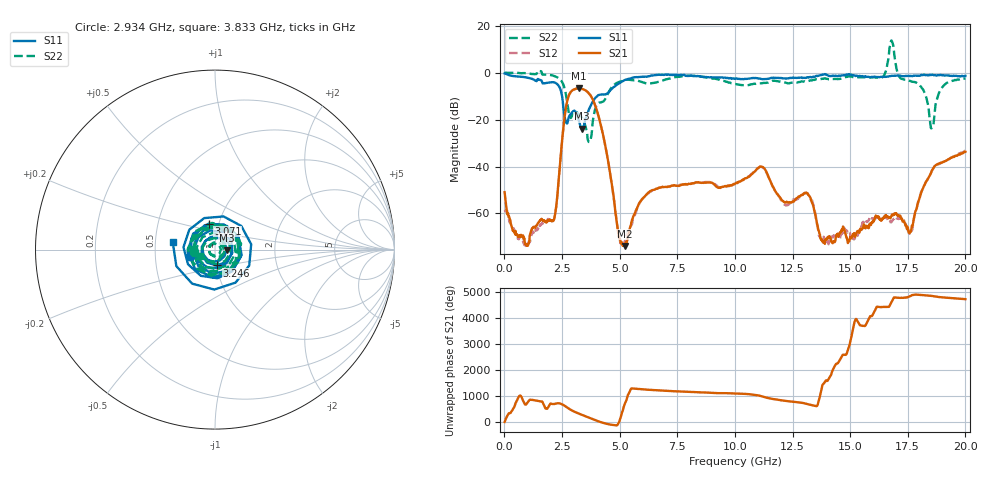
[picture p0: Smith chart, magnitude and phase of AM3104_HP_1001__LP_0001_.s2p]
!Created with skrf (http://scikit-rf.org).
# Hz S RI R 50.0
!freq ReS11 ImS11 ReS21 ImS21 ReS12 ImS12 ReS22 ImS22
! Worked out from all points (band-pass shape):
!   1601 points, 10 MHz to 20 GHz, reference 50 ohm
!   highest |S21| = -6.73 dB at 3.246 GHz (marker M1); lowest = -73.8 dB at 5.22 GHz (marker M2)
!   |S21| within 3 dB of the highest: 2.796 GHz to 3.741 GHz (944.9 MHz wide, 28.9 % of centre)
!   lowest |S11| = -23.8 dB at 3.346 GHz (marker M3), VSWR 1.14, Z = 56.9 - j0.37 ohm
!   |S11| at or under -10 dB: 2.502 GHz to 4.029 GHz (1.527 GHz wide, 46.8 % of centre)
!   |S22| runs from -29.6 to 13.7 dB; largest |S21 - S12| = 0.024
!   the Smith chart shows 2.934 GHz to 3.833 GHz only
!   S11 on the Smith chart (normalised r, x): 2.934 GHz: 0.76, -0.06; 3.071 GHz: 0.89, +0.26; 3.246 GHz: 1.00, -0.18; 3.833 GHz: 0.62, +0.05
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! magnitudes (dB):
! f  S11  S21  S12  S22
! 10 MHz  -0.3  -50.9  -58.4  0.0
! 972 MHz  -2.1  -73.2  -73.7  -0.2
! 2.109 GHz  -4.1  -63.2  -63.1  -1.2
! 2.646 GHz  -20.3  -16.5  -16.5  -8.1
! 2.934 GHz  -16.9  -7.7  -7.7  -18.4
! 3.071 GHz  -16.5  -7.0  -7.0  -16.5
! 3.246 GHz  -21.0  -6.7  -6.8  -18.1
! 3.346 GHz  -23.8  -6.9  -7.0  -18.9
! 3.833 GHz  -12.4  -11.4  -11.4  -20.9
! 5.22 GHz  -3.2  -73.8  -72.1  -3.2
! 6.682 GHz  -0.9  -49.2  -49.1  -3.9
! 10.01 GHz  -2.6  -47.4  -47.6  -4.9
! 11.17 GHz  -2.8  -40.1  -40.2  -4.5
! 12.15 GHz  -2.5  -55.2  -56.3  -4.2
! 13.34 GHz  -2.0  -55.1  -54.4  -3.3
! 13.99 GHz  -0.9  -71.1  -72.8  -2.7
! 16.35 GHz  -1.8  -63.1  -62.6  -2.3
! 16.68 GHz  -1.5  -62.0  -63.4  7.2
! 17.61 GHz  -1.4  -67.7  -69.0  -3.5
! 18.54 GHz  -0.9  -41.9  -42.1  -23.6
! 19 GHz  -1.2  -38.3  -38.2  -6.2
! 20 GHz  -1.4  -33.7  -33.3  -2.5
